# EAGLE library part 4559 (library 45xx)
8-bit SUCCESSIVE APPROXIMATION REGISTER
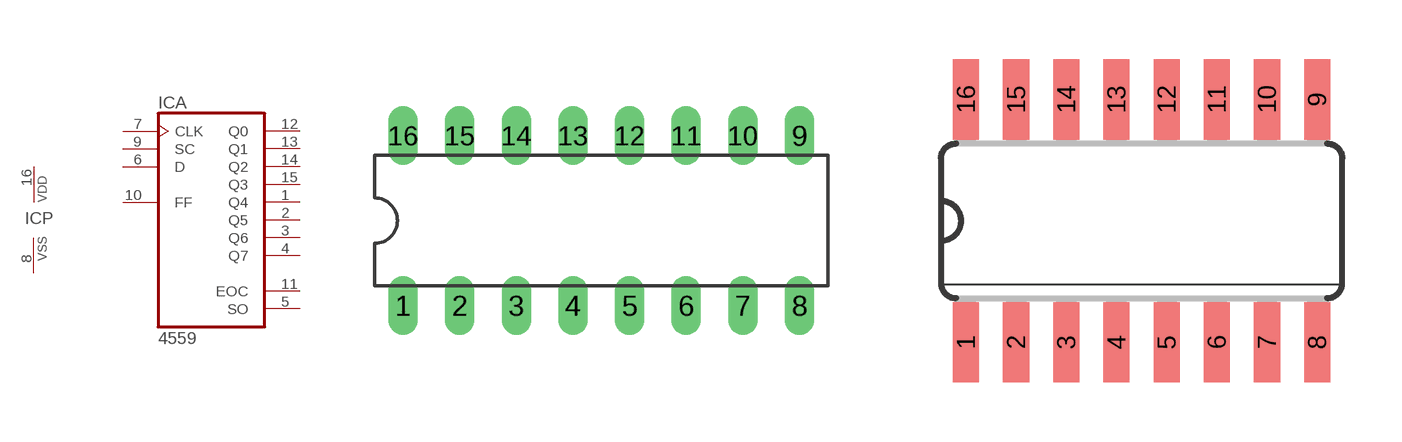
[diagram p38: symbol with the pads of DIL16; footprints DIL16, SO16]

Designator prefix IC; gates A=4559 P=PWRN

## 4559N  [DIL16]
1  A:Q4  out
2  A:Q5  out
3  A:Q6  out
4  A:Q7  out
5  A:SO  out
6  A:D  in
7  A:CLK  in
8  P:VSS  pwr
9  A:SC  in
10  A:FF  in
11  A:EOC  out
12  A:Q0  out
13  A:Q1  out
14  A:Q2  out
15  A:Q3  out
16  P:VDD  pwr

## 4559D  [SO16]
Pads as for DIL16

## Footprint DIL16 (pad centres in mm)
Dual In Line Package
drill 0.813 long: 1 -8.89,-3.81; 2 -6.35,-3.81; 3 -3.81,-3.81; 4 -1.27,-3.81; 5 1.27,-3.81; 6 3.81,-3.81; 7 6.35,-3.81; 8 8.89,-3.81; 9 8.89,3.81; 10 6.35,3.81; 11 3.81,3.81; 12 1.27,3.81; 13 -1.27,3.81; 14 -3.81,3.81; 15 -6.35,3.81; 16 -8.89,3.81

## Footprint SO16 (pad centres in mm)
Small Outline package 150 mil
smd 0.66 x 2.032: 1 -4.445,-3.073; 2 -3.175,-3.073; 3 -1.905,-3.073; 4 -0.635,-3.073; 5 0.635,-3.073; 6 1.905,-3.073; 7 3.175,-3.073; 8 4.445,-3.073; 9 4.445,3.073; 10 3.175,3.073; 11 1.905,3.073; 12 0.635,3.073; 13 -0.635,3.073; 14 -1.905,3.073; 15 -3.175,3.073; 16 -4.445,3.073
